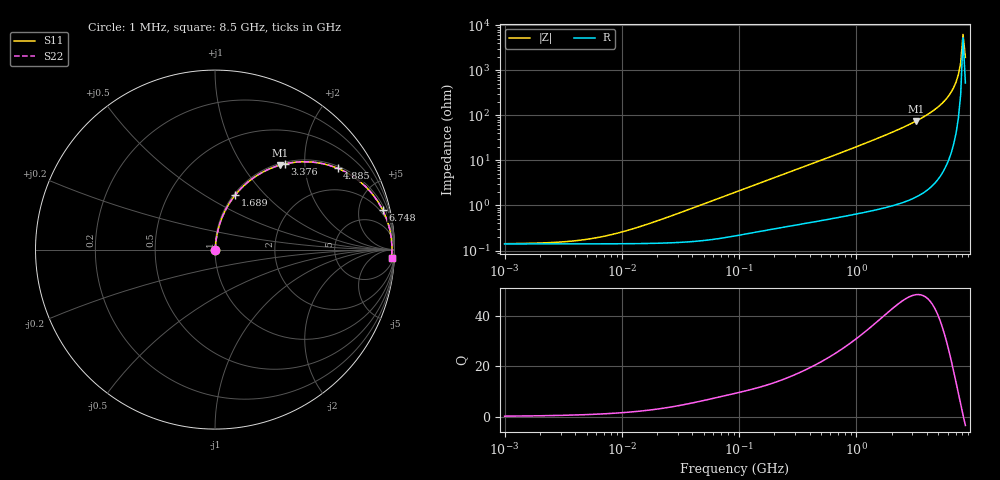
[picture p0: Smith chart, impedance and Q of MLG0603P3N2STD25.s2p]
! S-Parameter Data Generated by TDK Corporation
! Copyright(C) 2025 TDK Corporation.
! All Rights Reserved.
! TDK P/N: MLG0603P3N2STD25 (SMD / SMT Inductor (Coil))
! Property: L=3.2nH at 500MHz
! Size(LxWxT): 0.6x0.3x0.3mm
! Model Type: s2p (Touchstone File Format Version 1.0)
! Frequency: DC=Yes Start=1MHz Stop=8500MHz 198points Log-sweep
! Model Generated on Feb. 6, 2025
! Terms and conditions regarding TDK Simulation Models:
! 1)This simulation model is being provided solely for informational
!  purposes. Please refer to the specifications of the products in
!  terms of detailed characteristics of such products.
! 2)In no event shall TDK Corporation of any of its subsidiaries be
!  liable for any loss or damage arising, directly or indirectly,
!  from any information contained in this simulation model, including,
!  but not limited to loss or damages arising from any inaccuracies,
!  omissions or errors in connection with such information.
! 3)Any and all copyrights on this simulation model are owned by
!  TDK Corporation.  Duplication or redistribution of this simulation
!  model without prior written permission from TDK Corporation
!  is prohibited.
! 4)This simulation model is subject to any modification or change
!  without any prior notice.
! 5)Neither TDK Corporation nor any of its subsidiaries shall make any
!  warranty, express or implied, including but not limited to the
!  correctness, implied warranties of merchantability and fitness for
!  a particular purpose with respect to this simulation models.
! 6)The use of this simulation model shall be deemed to have consented
!  to the terms and conditions hereof.
! Port Assignments:
!  1 ---@@@--- 2
! Applicable Conditions:
!  Temperature = 25 degC
!  DC Bias Current = 0 A
!  Small Signal Operation
# Hz S MA R 50
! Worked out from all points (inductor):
!   197 points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, 1 MHz to 8.5 GHz, reference 50 ohm
!   read as one part in series: L = 3.43 nH near 21.05 MHz
!   highest Q = 48.7 at 3.224 GHz (marker M1), where L = 3.68 nH
!   self-resonance near 8.117 GHz
!   S11 on the Smith chart (normalised r, x): 1 MHz: 1.00, +0.00; 1.689 GHz: 1.02, +0.69; 3.376 GHz: 1.03, +1.59; 4.885 GHz: 1.07, +2.96; 6.748 GHz: 1.46, +8.24; 8.5 GHz: 11, -37
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1000000  0.001415 8.8  0.9986 -0.0  0.9986 -0.0  0.001415 8.8
2403882  0.001492 20.3  0.9986 -0.0  0.9986 -0.0  0.001492 20.3
4587603  0.001714 35.2  0.9986 -0.1  0.9986 -0.1  0.001714 35.2
9168677  0.002426 54.4  0.9986 -0.1  0.9986 -0.1  0.002426 54.4
2.10461e7  0.004754 72.0  0.9985 -0.3  0.9985 -0.3  0.004754 72.0
9.219544e7  0.0195 82.7  0.9977 -1.1  0.9977 -1.1  0.0195 82.7
4.229561e8  0.08469 82.3  0.9922 -4.9  0.9922 -4.9  0.08469 82.3
8.852465e8  0.1739 78.0  0.9788 -10.0  0.9788 -10.0  0.1739 78.0
1.689417e9  0.3253 69.6  0.9375 -19.0  0.9375 -19.0  0.3253 69.6
1.940355e9  0.3713 66.9  0.9198 -21.8  0.9198 -21.8  0.3713 66.9
2.559585e9  0.4814 60.0  0.8662 -28.8  0.8662 -28.8  0.4814 60.0
3.224109e9  0.5923 52.5  0.7936 -36.3  0.7936 -36.3  0.5923 52.5
3.37643e9  0.6165 50.8  0.7748 -38.0  0.7748 -38.0  0.6165 50.8
4.061159e9  0.7174 43.0  0.6816 -45.8  0.6816 -45.8  0.7174 43.0
4.884749e9  0.8198 33.6  0.5532 -55.0  0.5532 -55.0  0.8198 33.6
5.87536e9  0.9105 22.6  0.3843 -65.5  0.3843 -65.5  0.9105 22.6
6.748056e9  0.9598 13.4  0.2325 -73.4  0.2325 -73.4  0.9598 13.4
7.066863e9  0.9711 10.2  0.1783 -75.6  0.1783 -75.6  0.9711 10.2
7.400733e9  0.9795 7.0  0.1227 -76.9  0.1227 -76.9  0.9795 7.0
7.750377e9  0.9846 3.7  0.06671 -74.8  0.06671 -74.8  0.9846 3.7
8.116539e9  0.9865 0.5  0.01578 -30.9  0.01578 -30.9  0.9865 0.5
8.5e9  0.985 -2.8  0.05092 71.5  0.05092 71.5  0.985 -2.8
